| TEXAS INSTRUMENTS INCORPORATED
| Standard Linear and Logic Group
| IBIS Model of SN74ABT16240A
| 16-BIT BUFFERS/DRIVERS WITH 3-STATE OUTPUTS
| This file contains package information for the following:
|  TSSOP 48-pin (DGG) package as [Component] ABT16240A_DGG
|  TVSOP 48-pin (DGV) package as [Component] ABT16240A_DGV
|  SSOP 48-pin (DL) package as [Component] ABT16240A_DL
| This device can be powered at the following Vccs:
|  5 volt Vcc
| This file provides unique models under the [Model Selector] for each Vcc.
| For operation at a specific Vcc, select the appropriate model after each
| [Model Selector] keyword.
[IBIS Ver]   3.2
[Comment char]  |_char
[File Name]   sn74abt16240a.ibs
[File Rev]   1.1 | d_die
[Date]   August 16, 2001
[Source]   Data created from TI-SPICE simulations at TI-SLL.
[Notes]   The following is an IBIS list for the ABT16240A.
   Please contact sllibis@ti.com with questions and
   comments concerning SLL IBIS models.
   -This IBIS model is created from a BA (back annotated netlist
   Non-Convergence in the following files:
   pc_abt16240a_out, extrapolated from 5.445 V plus
   pu_abt16240a_out, extrapolated from 5.21 V plus
   pc_abt16240a_out, extrapolated from 5.445 V plus
   pu_abt16240a_out, extrapolated from 5.21 V plus
   gc_abt16240a_out, extrapolated from -0.445 V minus
   pd_abt16240a_out, extrapolated from -0.21 V minus
   -The non-monotonic warning is due to non-convergence
   -As there is no power clamp diode in the Input Model,
   we removed the Pwr Clamp table data from the Input Model
[Disclaimer] Property of Texas Instruments Incorporated.  Unauthorized
   reproduction and/or distribution is strictly prohibited.
   This product is protected under copyright law.
   Created  2001, (C) Copyright  2001, Texas Instruments
   Incorporated, All Rights Reserved
   UNLESS THERE IS A SIGNED, WRITTEN AGREEMENT TO THE
   CONTRARY, TEXAS INSTRUMENTS (TI) IS PROVIDING THE IBIS
   MODELS  AND WITHOUT ANY WARRANTY, EXPRESSED OR
   IMPLIED.  TI assumes no liability for:
   1) the accuracy of the IBIS models provided to your
   company;
   2) the proper functioning of these IBIS Models in your
   design or for any resulting applications; or
   3) infringement of patents, copyrights or intellectual
   property rights resulting from your use of these IBIS
   models.
   TI provides IBIS Models as a service to our customers.
   You and your company shall not distribute, sell or give
   these models to anyone else without prior written
   permission from TI.
   TI reserves the right to make changes to our products or
   to discontinue any semiconductor product or service
   without notice, and advises our customers to obtain the
   latest version of relevant information to verify, before
   placing orders, that the information being relied on is
   current.
   Please be aware that your receipt and use of the IBIS
   information provided shall serve as acceptance of these
   terms and conditions.  If you do not accept these terms,
   you should return or destroy the IBIS models and any
   other accompanying information immediately.
| Component ABT16240A_DGG 48-pin TSSOP
[Component]   ABT16240A_DGG
[Manufacturer]   Texas Instruments, Inc.
[Package]
|   typ   min   max
R_pkg   4.400e-02   3.800e-02   5.100e-02
L_pkg   3.019e-09   2.486e-09   4.099e-09
C_pkg   5.070e-13   3.340e-13   8.090e-13
[Pin]   signal_name   model_name   R_pin   L_pin   C_pin
1   1NOE   ABT16240A_NOE   4.100e-02   4.017e-09   7.590e-13
2   1Y1   ABT16240A_OUT   4.200e-02   3.737e-09   7.920e-13
3   1Y2   ABT16240A_OUT   4.200e-02   3.480e-09   6.610e-13
4   GND   GND   3.800e-02   3.131e-09   5.750e-13
5   1Y3   ABT16240A_OUT   4.700e-02   3.122e-09   5.660e-13
6   1Y4   ABT16240A_OUT   4.300e-02   2.948e-09   5.040e-13
7   VCC   POWER   4.500e-02   2.845e-09   3.970e-13
8   2Y1   ABT16240A_OUT   4.900e-02   2.835e-09   3.940e-13
9   2Y2   ABT16240A_OUT   4.800e-02   2.715e-09   3.780e-13
10   GND   GND   5.000e-02   2.664e-09   3.630e-13
11   2Y3   ABT16240A_OUT   5.000e-02   2.585e-09   3.480e-13
12   2Y4   ABT16240A_OUT   4.900e-02   2.550e-09   3.370e-13
13   3Y1   ABT16240A_OUT   4.900e-02   2.541e-09   3.360e-13
14   3Y2   ABT16240A_OUT   5.000e-02   2.574e-09   3.480e-13
15   GND   GND   4.900e-02   2.618e-09   3.590e-13
16   3Y3   ABT16240A_OUT   4.600e-02   2.671e-09   3.750e-13
17   3Y4   ABT16240A_OUT   4.500e-02   2.754e-09   3.890e-13
18   VCC   POWER   4.400e-02   2.823e-09   4.500e-13
19   4Y1   ABT16240A_OUT   4.200e-02   2.968e-09   5.030e-13
20   4Y2   ABT16240A_OUT   5.100e-02   3.108e-09   5.350e-13
21   GND   GND   4.200e-02   3.175e-09   5.870e-13
22   4Y3   ABT16240A_OUT   4.100e-02   3.449e-09   6.780e-13
23   4Y4   ABT16240A_OUT   4.400e-02   3.766e-09   8.040e-13
24   4NOE   ABT16240A_NOE   4.300e-02   4.065e-09   7.610e-13
25   3NOE   ABT16240A_NOE   4.100e-02   3.994e-09   7.570e-13
26   4A4   ABT16240A_IN   3.900e-02   3.649e-09   7.890e-13
27   4A3   ABT16240A_IN   3.800e-02   3.362e-09   6.600e-13
28   GND   GND   3.800e-02   3.082e-09   5.740e-13
29   4A2   ABT16240A_IN   4.400e-02   2.990e-09   5.220e-13
30   4A1   ABT16240A_IN   4.100e-02   2.917e-09   4.950e-13
31   VCC   POWER   4.300e-02   2.820e-09   4.480e-13
32   3A4   ABT16240A_IN   4.300e-02   2.699e-09   3.850e-13
33   3A3   ABT16240A_IN   4.500e-02   2.628e-09   3.720e-13
34   GND   GND   4.600e-02   2.556e-09   3.560e-13
35   3A2   ABT16240A_IN   4.600e-02   2.495e-09   3.440e-13
36   3A1   ABT16240A_IN   4.700e-02   2.487e-09   3.340e-13
37   2A4   ABT16240A_IN   4.700e-02   2.490e-09   3.350e-13
38   2A3   ABT16240A_IN   4.600e-02   2.486e-09   3.430e-13
39   GND   GND   4.500e-02   2.566e-09   3.560e-13
40   2A2   ABT16240A_IN   4.400e-02   2.639e-09   3.740e-13
41   2A1   ABT16240A_IN   4.300e-02   2.701e-09   3.860e-13
42   VCC   POWER   4.300e-02   2.817e-09   4.500e-13
43   1A4   ABT16240A_IN   4.100e-02   2.935e-09   5.010e-13
44   1A3   ABT16240A_IN   4.700e-02   3.035e-09   5.290e-13
45   GND   GND   4.300e-02   3.171e-09   5.890e-13
46   1A2   ABT16240A_IN   4.000e-02   3.415e-09   6.820e-13
47   1A1   ABT16240A_IN   4.300e-02   3.741e-09   8.090e-13
48   2NOE   ABT16240A_NOE   4.400e-02   4.099e-09   7.640e-13
| Component ABT16240A_DGV 48-pin TVSOP
[Component]   ABT16240A_DGV
[Manufacturer]   Texas Instruments, Inc.
[Package]
|   typ   min   max
R_pkg   7.000e-02   4.900e-02   8.500e-02
L_pkg   3.013e-09   2.743e-09   3.408e-09
C_pkg   3.710e-13   2.940e-13   5.110e-13
[Pin]   signal_name   model_name   R_pin   L_pin   C_pin
1   1NOE   ABT16240A_NOE   4.900e-02   3.393e-09   4.970e-13
2   1Y1   ABT16240A_OUT   6.000e-02   3.250e-09   5.020e-13
3   1Y2   ABT16240A_OUT   7.700e-02   3.310e-09   4.510e-13
4   GND   GND   8.500e-02   3.299e-09   4.040e-13
5   1Y3   ABT16240A_OUT   8.300e-02   3.136e-09   3.600e-13
6   1Y4   ABT16240A_OUT   7.700e-02   3.019e-09   3.630e-13
7   VCC   POWER   6.500e-02   2.882e-09   3.490e-13
8   2Y1   ABT16240A_OUT   6.600e-02   2.829e-09   3.140e-13
9   2Y2   ABT16240A_OUT   6.700e-02   2.796e-09   3.140e-13
10   GND   GND   6.900e-02   2.754e-09   3.080e-13
11   2Y3   ABT16240A_OUT   7.000e-02   2.753e-09   3.010e-13
12   2Y4   ABT16240A_OUT   7.100e-02   2.745e-09   2.940e-13
13   3Y1   ABT16240A_OUT   7.000e-02   2.744e-09   2.940e-13
14   3Y2   ABT16240A_OUT   7.000e-02   2.754e-09   3.010e-13
15   GND   GND   6.900e-02   2.754e-09   3.080e-13
16   3Y3   ABT16240A_OUT   6.700e-02   2.796e-09   3.140e-13
17   3Y4   ABT16240A_OUT   6.600e-02   2.829e-09   3.140e-13
18   VCC   POWER   6.500e-02   2.883e-09   3.500e-13
19   4Y1   ABT16240A_OUT   7.500e-02   3.014e-09   3.630e-13
20   4Y2   ABT16240A_OUT   8.000e-02   3.128e-09   3.580e-13
21   GND   GND   8.400e-02   3.295e-09   4.030e-13
22   4Y3   ABT16240A_OUT   7.800e-02   3.311e-09   4.520e-13
23   4Y4   ABT16240A_OUT   6.200e-02   3.259e-09   5.010e-13
24   4NOE   ABT16240A_NOE   5.200e-02   3.404e-09   4.960e-13
25   3NOE   ABT16240A_NOE   5.300e-02   3.397e-09   5.050e-13
26   4A4   ABT16240A_IN   6.200e-02   3.249e-09   5.110e-13
27   4A3   ABT16240A_IN   7.700e-02   3.308e-09   4.530e-13
28   GND   GND   8.200e-02   3.289e-09   4.030e-13
29   4A2   ABT16240A_IN   7.800e-02   3.121e-09   3.590e-13
30   4A1   ABT16240A_IN   7.400e-02   3.010e-09   3.630e-13
31   VCC   POWER   6.500e-02   2.883e-09   3.490e-13
32   3A4   ABT16240A_IN   6.700e-02   2.829e-09   3.140e-13
33   3A3   ABT16240A_IN   6.700e-02   2.795e-09   3.140e-13
34   GND   GND   6.900e-02   2.753e-09   3.070e-13
35   3A2   ABT16240A_IN   7.000e-02   2.753e-09   3.010e-13
36   3A1   ABT16240A_IN   7.000e-02   2.743e-09   2.940e-13
37   2A4   ABT16240A_IN   7.000e-02   2.743e-09   2.940e-13
38   2A3   ABT16240A_IN   7.000e-02   2.753e-09   3.010e-13
39   GND   GND   6.900e-02   2.754e-09   3.070e-13
40   2A2   ABT16240A_IN   6.800e-02   2.797e-09   3.140e-13
41   2A1   ABT16240A_IN   6.700e-02   2.830e-09   3.140e-13
42   VCC   POWER   6.400e-02   2.880e-09   3.490e-13
43   1A4   ABT16240A_IN   7.200e-02   3.004e-09   3.620e-13
44   1A3   ABT16240A_IN   7.800e-02   3.121e-09   3.590e-13
45   GND   GND   8.400e-02   3.296e-09   4.030e-13
46   1A2   ABT16240A_IN   7.700e-02   3.308e-09   4.510e-13
47   1A1   ABT16240A_IN   6.200e-02   3.258e-09   4.990e-13
48   2NOE   ABT16240A_NOE   5.300e-02   3.408e-09   4.940e-13
| Component ABT16240A_DL 48-pin SSOP
[Component]   ABT16240A_DL
[Manufacturer]   Texas Instruments, Inc.
[Package]
|   typ   min   max
R_pkg   4.800e-02   3.800e-02   5.300e-02
L_pkg   6.046e-09   5.084e-09   7.968e-09
C_pkg   8.130e-13   5.690e-13   1.157e-12
[Pin]   signal_name   model_name   R_pin   L_pin   C_pin
1   1NOE   ABT16240A_NOE   4.600e-02   7.968e-09   1.017e-12
2   1Y1   ABT16240A_OUT   4.400e-02   7.299e-09   1.157e-12
3   1Y2   ABT16240A_OUT   4.300e-02   6.765e-09   1.058e-12
4   GND   GND   4.100e-02   6.269e-09   9.330e-13
5   1Y3   ABT16240A_OUT   3.800e-02   5.856e-09   8.290e-13
6   1Y4   ABT16240A_OUT   4.600e-02   5.802e-09   7.900e-13
7   VCC   POWER   5.000e-02   5.656e-09   7.380e-13
8   2Y1   ABT16240A_OUT   5.300e-02   5.500e-09   6.430e-13
9   2Y2   ABT16240A_OUT   5.200e-02   5.304e-09   6.060e-13
10   GND   GND   5.300e-02   5.189e-09   5.830e-13
11   2Y3   ABT16240A_OUT   5.100e-02   5.084e-09   5.690e-13
12   2Y4   ABT16240A_OUT   5.300e-02   5.862e-09   8.330e-13
13   3Y1   ABT16240A_OUT   5.300e-02   5.862e-09   8.330e-13
14   3Y2   ABT16240A_OUT   5.100e-02   5.084e-09   5.690e-13
15   GND   GND   5.300e-02   5.189e-09   5.830e-13
16   3Y3   ABT16240A_OUT   5.200e-02   5.304e-09   6.060e-13
17   3Y4   ABT16240A_OUT   5.300e-02   5.500e-09   6.430e-13
18   VCC   POWER   5.000e-02   5.656e-09   7.380e-13
19   4Y1   ABT16240A_OUT   4.600e-02   5.802e-09   7.900e-13
20   4Y2   ABT16240A_OUT   3.800e-02   5.856e-09   8.290e-13
21   GND   GND   4.100e-02   6.269e-09   9.330e-13
22   4Y3   ABT16240A_OUT   4.300e-02   6.765e-09   1.058e-12
23   4Y4   ABT16240A_OUT   4.400e-02   7.299e-09   1.157e-12
24   4NOE   ABT16240A_NOE   4.600e-02   7.968e-09   1.017e-12
25   3NOE   ABT16240A_NOE   4.600e-02   7.968e-09   1.017e-12
26   4A4   ABT16240A_IN   4.400e-02   7.299e-09   1.157e-12
27   4A3   ABT16240A_IN   4.300e-02   6.765e-09   1.058e-12
28   GND   GND   4.100e-02   6.269e-09   9.330e-13
29   4A2   ABT16240A_IN   3.800e-02   5.856e-09   8.290e-13
30   4A1   ABT16240A_IN   4.600e-02   5.802e-09   7.900e-13
31   VCC   POWER   5.000e-02   5.656e-09   7.380e-13
32   3A4   ABT16240A_IN   5.300e-02   5.500e-09   6.430e-13
33   3A3   ABT16240A_IN   5.200e-02   5.304e-09   6.060e-13
34   GND   GND   5.300e-02   5.189e-09   5.830e-13
35   3A2   ABT16240A_IN   5.100e-02   5.084e-09   5.690e-13
36   3A1   ABT16240A_IN   5.300e-02   5.862e-09   8.330e-13
37   2A4   ABT16240A_IN   5.300e-02   5.862e-09   8.330e-13
38   2A3   ABT16240A_IN   5.100e-02   5.084e-09   5.690e-13
39   GND   GND   5.300e-02   5.189e-09   5.830e-13
40   2A2   ABT16240A_IN   5.200e-02   5.304e-09   6.060e-13
41   2A1   ABT16240A_IN   5.300e-02   5.500e-09   6.430e-13
42   VCC   POWER   5.000e-02   5.656e-09   7.380e-13
43   1A4   ABT16240A_IN   4.600e-02   5.802e-09   7.900e-13
44   1A3   ABT16240A_IN   3.800e-02   5.856e-09   8.290e-13
45   GND   GND   4.100e-02   6.269e-09   9.330e-13
46   1A2   ABT16240A_IN   4.300e-02   6.765e-09   1.058e-12
47   1A1   ABT16240A_IN   4.400e-02   7.299e-09   1.157e-12
48   2NOE   ABT16240A_NOE   4.600e-02   7.967e-09   1.017e-12
| Models and submodels in the file (3): ABT16240A_IN (Input), ABT16240A_NOE (Input), ABT16240A_OUT (3-state)
